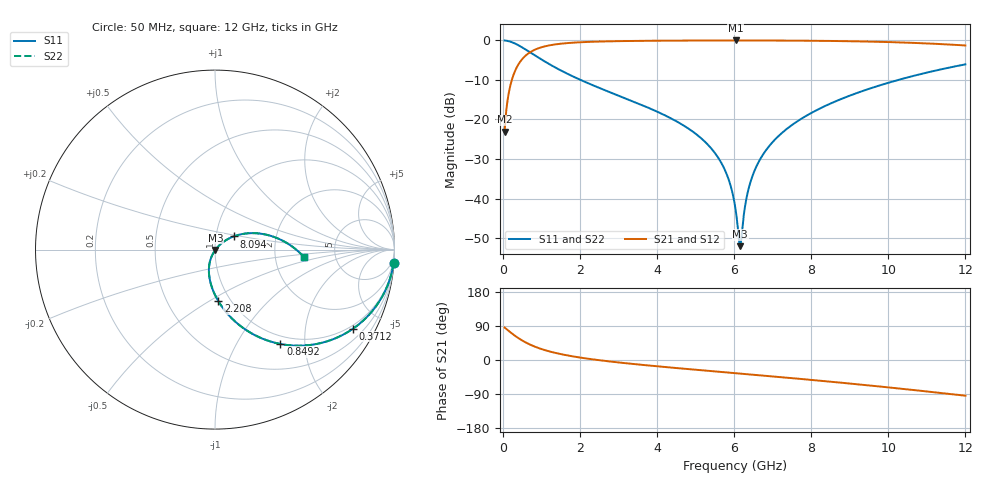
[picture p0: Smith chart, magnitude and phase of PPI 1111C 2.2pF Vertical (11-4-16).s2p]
# GHz S MA R 50
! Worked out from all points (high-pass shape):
!   1601 points, 50 MHz to 12 GHz, reference 50 ohm
!   highest |S21| = -0.02 dB at 6.047 GHz (marker M1); lowest = -23.1 dB at 50 MHz (marker M2)
!   |S21| within 3 dB of the highest: 707.6 MHz to end of sweep
!   lowest |S11| = -52.0 dB at 6.159 GHz (marker M3), VSWR 1.01, Z = 50.2 - j0.137 ohm
!   |S11| at or under -10 dB: 2.02 GHz to 10.26 GHz (8.241 GHz wide, 134 % of centre)
!   |S22| runs from -52.0 to 0.0 dB; largest |S21 - S12| = 0
!   S11 on the Smith chart (normalised r, x): 50 MHz: 1, -27; 371.2 MHz: 0.87, -3.57; 849.2 MHz: 0.87, -1.54; 2.208 GHz: 0.88, -0.55; 8.094 GHz: 1.22, +0.18; 12 GHz: 2.94, -0.32
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0.05  0.9975 -4.3  0.06992 85.7  0.06992 85.7  0.9975 -4.3
0.1919063  0.9656 -16.2  0.2599 73.8  0.2599 73.8  0.9656 -16.2
0.3711563  0.8866 -29.8  0.462 60.2  0.462 60.2  0.8866 -29.8
0.8491562  0.6395 -55.3  0.7679 34.6  0.7679 34.6  0.6395 -55.3
1.349562  0.4584 -70.7  0.8875 19.1  0.8875 19.1  0.4584 -70.7
2.044156  0.3124 -83.9  0.9484 5.9  0.9484 5.9  0.3124 -83.9
2.208469  0.2882 -86.3  0.956 3.5  0.956 3.5  0.2882 -86.3
4.038312  0.1235 -106.0  0.9902 -16.9  0.9902 -16.9  0.1235 -106.0
4.874812  0.07341 -112.9  0.9949 -24.6  0.9949 -24.6  0.07341 -112.9
5.442437  0.04119 -116.4  0.9966 -29.6  0.9966 -29.6  0.04119 -116.4
5.808406  0.0204 -116.1  0.9971 -32.8  0.9971 -32.8  0.0204 -116.1
6.025  0.008123 -107.1  0.9972 -34.7  0.9972 -34.7  0.008123 -107.1
6.047406  0.006893 -103.9  0.9972 -34.9  0.9972 -34.9  0.006893 -103.9
6.114625  0.003531 -80.7  0.9972 -35.5  0.9972 -35.5  0.003531 -80.7
6.159438  0.002504 -33.0  0.9972 -35.9  0.9972 -35.9  0.002504 -33.0
6.3835  0.01368 41.3  0.997 -37.9  0.997 -37.9  0.01368 41.3
6.68225  0.03175 44.7  0.9965 -40.5  0.9965 -40.5  0.03175 44.7
7.212531  0.06562 42.2  0.9946 -45.2  0.9946 -45.2  0.06562 42.2
8.019156  0.122 35.8  0.9889 -52.7  0.9889 -52.7  0.122 35.8
8.093844  0.1276 35.2  0.9882 -53.4  0.9882 -53.4  0.1276 35.2
10.01331  0.2921 16.8  0.9518 -72.4  0.9518 -72.4  0.2921 16.8
12  0.4977 -4.8  0.8616 -94.2  0.8616 -94.2  0.4977 -4.8
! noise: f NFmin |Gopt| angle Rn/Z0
0.05  0.0006793  0.9419  2.227  0.002614
1.372  0.004114  0.7008  10.16  0.002672
2.701  0.006459  0.6408  17.58  0.003321
4.031  0.008566  0.6108  24.86  0.003904
5.36  0.01061  0.5971  31.85  0.0045
6.682  0.01268  0.5945  38.44  0.005158
8.012  0.01487  0.6006  44.68  0.005933
9.341  0.01725  0.6139  50.55  0.006876
10.67  0.01991  0.633  56.08  0.008062
12  0.02295  0.6571  61.32  0.009591
